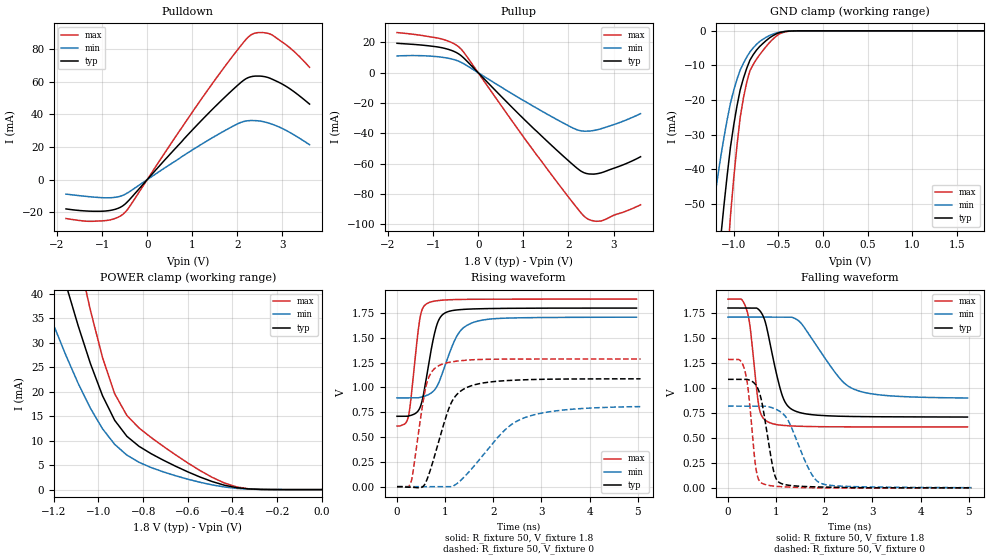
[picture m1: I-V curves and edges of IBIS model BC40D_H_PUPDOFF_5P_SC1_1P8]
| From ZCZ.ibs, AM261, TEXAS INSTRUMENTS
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|BC40D_H_PU_ON_10P_SC1_3P3; BUFFER WITH WEAK_PULLUP_ON AT 10% SUPPLY
|VARIATION WITH SC1=1 MEANING SLOW MODE OF OPERATION
|   Model Cell BC40D_H_PUPDOFF_5P_SC1_1P8
|BC40D_H_PUPDOFF_5P_SC1_1P8
[Model]   BC40D_H_PUPDOFF_5P_SC1_1P8
Model_type   I/O
Polarity   Non-Inverting
Enable   Active-Low
Vinl =  0.63
Vinh =  1.17
Cref =  15pF
Rref =  100.0000M
Vref =  0V
Vmeas =  0.9
C_comp   2.364487p   2.290698p   2.389419p
|[Input load] weak_pupdoff
|[Output drive] slow
|[supplytol] 5
|[temp] ind
[Model Spec]
Vinl   0.63   0.5985   0.6615
Vinh   1.17   1.1115   1.2285
[Temperature Range]   25   125   -40
[Voltage Range]   1.8   1.71   1.89
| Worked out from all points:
|   slope of the pulldown table from 0 to 0.27 V, typ, clamps not added: 32.2 ohm
|   slope of the pullup table from 0 to 0.27 V, typ, clamps not added: 32.6 ohm
|   GND clamp passes 1 mA (typ) near -0.53 V on its own axis
|   POWER clamp passes 1 mA (typ) near -0.44 V on its own axis
|   rising waveform, R_fixture 50, V_fixture 1.8: 20-80 % time 249ps typ, 403ps min, 171ps max; typ from 0.709 V to 1.8 V
|   rising waveform, R_fixture 50, V_fixture 0: 20-80 % time 430ps typ, 919ps min, 247ps max; typ from 0 V to 1.09 V
|   falling waveform, R_fixture 50, V_fixture 1.8: 20-80 % time 311ps typ, 721ps min, 173ps max; typ from 1.8 V to 0.709 V
|   falling waveform, R_fixture 50, V_fixture 0: 20-80 % time 228ps typ, 434ps min, 155ps max; typ from 1.09 V to 0 V
| Nom Voltages:
|   VDD=1.1, VDDS=1.8, VDDS18=1.8, ESD_BIASFET=0, VSS=0, VSSS=0
| Min Voltages:
|   VDD=1.045, VDDS=1.71, VDDS18=1.71, ESD_BIASFET=0, VSS=0, VSSS=0
| Max Voltages:
|   VDD=1.16, VDDS=1.89, VDDS18=1.89, ESD_BIASFET=0, VSS=0, VSSS=0
[POWER_clamp]
|   voltage   I(typ)   I(min)   I(max)
-1.8V     158.8mA    112.5mA    219.7mA
-1.255V   59.93mA    39.99mA    84.86mA
-1.127V   39.08mA    25.5mA     55.75mA
-1.055V   28.36mA    18.34mA    40.41mA
-981.8mV  19.18mA    12.43mA    26.98mA
-927.3mV  14.16mA    9.239mA    19.58mA
-872.7mV  10.89mA    7.049mA    15.14mA
-818.2mV  8.843mA    5.579mA    12.59mA
-600mV    3.63mA     2.128mA    5.45mA
-436.4mV  903.9uA    539uA      1.358mA
-327.3mV  138.2uA    94.87uA    160.3uA
0V        19.3nA     133.7nA    230.3nA
[Pulldown]
|   voltage   I(typ)   I(min)   I(max)
-1.8V     -17.92mA   -8.85mA    -23.8mA
-1.309V   -19.26mA   -10.37mA   -25.5mA
-927.3mV  -19.22mA   -11.12mA   -25.08mA
-654.5mV  -17.65mA   -10.56mA   -23.13mA
-490.9mV  -14.97mA   -8.985mA   -20.05mA
1.364V    40.78mA    24.32mA    55.7mA
2.073V    59.41mA    35mA       81.91mA
2.291V    62.96mA    36.2mA     88.48mA
2.564V    63.25mA    35.58mA    90.07mA
2.782V    61.38mA    33.82mA    88.42mA
3.218V    54.59mA    28.02mA    79.45mA
3.6V      46.26mA    21.39mA    68.79mA
[Pullup]
|   voltage   I(typ)   I(min)   I(max)
-1.8V     19.42mA    11.07mA    26.5mA
-818.2mV  16.58mA    10.3mA     22.34mA
-545.5mV  14.19mA    8.748mA    19.29mA
-381.8mV  11.34mA    6.915mA    15.7mA
1.255V    -37.51mA   -22.64mA   -52.53mA
2.127V    -61.34mA   -36.82mA   -86.78mA
2.291V    -65.12mA   -38.38mA   -92.82mA
2.4V      -66.46mA   -38.53mA   -95.91mA
2.564V    -66.86mA   -38.08mA   -97.75mA
2.727V    -65.99mA   -36.9mA    -97.78mA
3.273V    -60.01mA   -31.26mA   -91.34mA
3.6V      -55.4mA    -26.98mA   -87.12mA
[GND_clamp]
|   voltage   I(typ)   I(min)   I(max)
-1.8V     -270.2mA   -170.2mA   -430.1mA
-1.255V   -91.66mA   -55.91mA   -148.4mA
-1.145V   -59.91mA   -36.45mA   -97.09mA
-1.109V   -50.48mA   -30.83mA   -81.55mA
-1.073V   -41.73mA   -25.65mA   -67.05mA
-1.036V   -33.66mA   -20.92mA   -53.59mA
-927.3mV  -17.07mA   -11.35mA   -25.04mA
-854.5mV  -10.86mA   -7.617mA   -14.91mA
-781.8mV  -6.919mA   -4.945mA   -9.771mA
-636.4mV  -2.823mA   -1.868mA   -4.529mA
-381.8mV  -84.73uA   -78.82uA   -126.1uA
1.8V      19.3nA     350.9nA    215.8nA
[Ramp]
| variable   typ   min   max
dV/dt_f 0.66158749/0.31320911n  0.4965113/0.73778172n 0.77345173/0.17433349n
dV/dt_r 0.65950744/0.43330442n 0.50319012/0.96393253n 0.77802263/0.24810359n
R_load = 50
[Rising Waveform]
R_fixture = 50
V_fixture = 1.8
V_fixture_min = 1.71
V_fixture_max = 1.89
|   time   V(typ)   V(min)   V(max)
0s        709.2mV    894.5mV    611.3mV
234.3ps   711.2mV    894.5mV    702.8mV
473.9ps   792.6mV    898.5mV    1.69V
534.4ps   892.2mV    906.1mV    1.799V
636.4ps   1.173V     924mV      1.849V
778.8ps   1.544V     974.5mV    1.87V
901.9ps   1.709V     1.09V      1.878V
1.242ns   1.781V     1.517V     1.886V
1.572ns   1.791V     1.653V     1.889V
4.974ns   1.8V       1.708V     1.89V
[Rising Waveform]
R_fixture = 50
V_fixture = 0
V_fixture_min = 0
V_fixture_max = 0
|   time   V(typ)   V(min)   V(max)
0s        0V         0V         0V
285.8ps   -5.093mV   0V         39.78mV
598.4ps   44.3mV     0V         1.004V
700.6ps   181mV      0V         1.142V
866.7ps   456.3mV    0V         1.219V
1.159ns   873.6mV    2.739mV    1.259V
1.555ns   1.019V     182.3mV    1.279V
2.25ns    1.068V     575.2mV    1.286V
2.653ns   1.077V     695.7mV    1.286V
5.059ns   1.087V     806.4mV    1.286V
[Falling Waveform]
R_fixture = 50
V_fixture = 1.8
V_fixture_min = 1.71
V_fixture_max = 1.89
|   time   V(typ)   V(min)   V(max)
0s        1.801V     1.71V      1.89V
275.2ps   1.801V     1.71V      1.89V
381.3ps   1.801V     1.71V      1.792V
462.6ps   1.801V     1.71V      1.598V
644.5ps   1.782V     1.71V      809.1mV
817.9ps   1.574V     1.71V      663.3mV
1.125ns   926.9mV    1.71V      626.1mV
1.384ns   771.4mV    1.697V     618.3mV
2.587ns   714.5mV    994mV      610.4mV
4.974ns   709mV      899.8mV    610mV
[Falling Waveform]
R_fixture = 50
V_fixture = 0
V_fixture_min = 0
V_fixture_max = 0
|   time   V(typ)   V(min)   V(max)
0s        1.086V     818.3mV    1.286V
345.5ps   1.086V     818.3mV    1.181V
422ps     1.083V     818.3mV    969.6mV
577.5ps   1.03V      818.3mV    200.5mV
706.3ps   848.9mV    818.3mV    45.77mV
946.7ps   169.4mV    797.1mV    17.7mV
1.102ns   44.25mV    757.3mV    11.8mV
1.724ns   11.16mV    148.6mV    0V
1.932ns   8.441mV    44.99mV    0V
5.059ns   0V         2.313mV    0V
